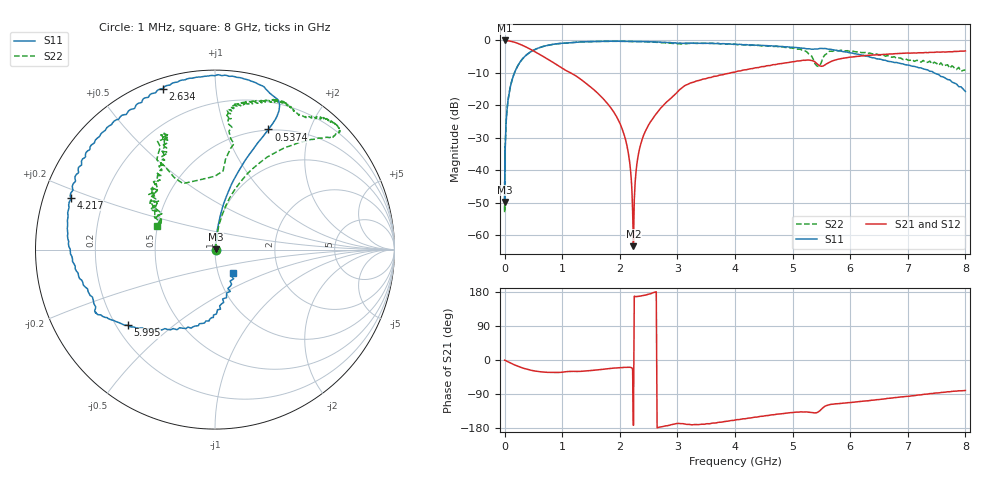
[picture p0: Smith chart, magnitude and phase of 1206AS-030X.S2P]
!s-Parameter Generated by FASTRON Sdn. Bhd.
!FASTRON P/N : 1206AS-030X
!Keysight Technologies: E5071C_MY46733604_B.14.02
!Date: Wed Nov 15 09:55:04 2023
!Version  :Rev00  Wed Nov 15 09:55:04 2023
!Data & Calibration Information:
!Freq  S11:SOLT2(ON)  S21:SOLT2(ON)  S12:SOLT2(ON)  S22:SOLT2(ON)
!PortZ  Port1:50+j0  Port2:50+j0
!When reading reference impedance value at option line is always used.
! Remarks : This data is being provided solely for informational purposes.
# Hz S dB R 50
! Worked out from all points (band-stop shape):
!   1601 points, 1 MHz to 8 GHz, reference 50 ohm
!   highest |S21| = -0.01 dB at 6.301 MHz (marker M1); lowest = -63.3 dB at 2.237 GHz (marker M2)
!   |S21| within 3 dB of the highest: start of sweep to 480.1 MHz
!   lowest |S11| = -49.7 dB at 1.505 MHz (marker M3), VSWR 1.01, Z = 50.3 + j0.0879 ohm
!   |S11| at or under -10 dB: start of sweep to 171.5 MHz; 7.458 GHz to end of sweep
!   |S22| runs from -53.0 to -0.3 dB; largest |S21 - S12| = 0.0068
!   S11 on the Smith chart (normalised r, x): 1 MHz: 1.01, -0.00; 537.4 MHz: 0.49, +1.42; 2.634 GHz: 0.04, +0.73; 4.217 GHz: 0.08, +0.17; 5.995 GHz: 0.25, -0.35; 8 GHz: 1.17, -0.32
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1000000  -47.00 -5.4  -0.03 -0.2  -0.04 -0.2  -48.63 -2.6
1504644  -49.71 15.5  -0.03 -0.2  -0.04 -0.2  -48.38 -2.7
4479405  -40.15 64.9  -0.04 -0.4  -0.04 -0.4  -40.44 68.6
6301378  -37.43 60.8  -0.01 -0.7  -0.06 -0.7  -40.41 70.4
2.00676e7  -27.87 81.5  -0.05 -1.7  -0.06 -1.6  -27.68 80.8
8.994653e7  -15.14 81.5  -0.20 -7.1  -0.21 -7.1  -15.19 79.3
4.006501e8  -4.17 68.7  -2.27 -25.0  -2.28 -25.0  -4.18 59.1
5.373938e8  -2.71 66.1  -3.58 -29.3  -3.59 -29.3  -2.72 53.1
1.225806e9  -0.57 72.2  -10.75 -30.2  -10.76 -30.3  -0.58 43.5
1.7949e9  -0.28 85.2  -19.59 -23.1  -19.61 -23.3  -0.28 44.9
2.029254e9  -0.26 91.3  -26.65 -20.2  -26.68 -20.5  -0.27 46.0
2.167736e9  -0.30 95.2  -36.90 -19.2  -36.93 -19.4  -0.30 47.8
2.237469e9  -0.32 97.2  -63.33 -172.4  -63.71 -171.9  -0.34 47.8
2.325502e9  -0.34 99.7  -34.89 167.9  -34.91 167.7  -0.37 48.6
2.44288e9  -0.38 102.7  -28.01 171.1  -28.05 170.8  -0.41 49.4
2.63362e9  -0.51 107.9  -22.59 179.9  -22.62 179.7  -0.58 51.0
3.162936e9  -0.84 125.7  -13.65 -169.9  -13.67 -170.0  -0.99 60.6
4.216915e9  -1.36 160.2  -8.93 -153.7  -8.91 -153.8  -1.38 76.0
5.192391e9  -2.39 -164.8  -6.11 -137.3  -6.07 -137.4  -3.22 82.3
5.668252e9  -2.75 -149.4  -6.49 -117.0  -6.46 -117.4  -3.32 118.0
5.995147e9  -3.82 -139.1  -5.14 -112.4  -5.12 -112.7  -3.42 113.3
8e9  -15.72 -53.0  -3.23 -80.3  -3.21 -80.8  -9.09 157.9
